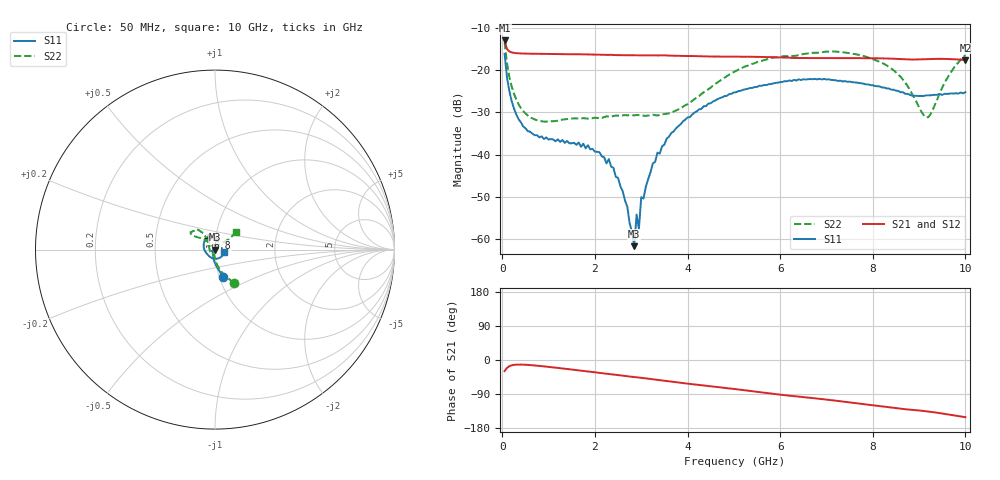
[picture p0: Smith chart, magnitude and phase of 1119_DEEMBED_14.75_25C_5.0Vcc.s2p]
!Hittite Microwave Corp.
!Digital Attenuator/PhaseShifter Rev 1.4.0
!Filename: C:\DATA\DATA\1119_DEEMBED_14.75_25C_5.0Vcc.s2p
!VNA ID: Agilent Technologies,N5224A,MY51441122,A.10.45.03
!Device type:
!2 Port Calibration.
!Temp(C): 25
!Lot Number:
!Serial Number:
!Operator:
!Misc:
!Attenuator:  14.750
# GHZ S DB R 50.0
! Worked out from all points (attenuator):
!   200 points, 50 MHz to 10 GHz, reference 50 ohm
!   highest |S21| = -12.92 dB at 50 MHz (marker M1); lowest = -17.6 dB at 10 GHz (marker M2)
!   lowest |S11| = -61.7 dB at 2.85 GHz (marker M3), VSWR 1.00, Z = 50 - j0.0816 ohm
!   |S11| at or under -10 dB: start of sweep to end of sweep
!   |S22| runs from -32.2 to -13.3 dB; largest |S21 - S12| = 0.00052
!   S11 on the Smith chart (normalised r, x): 50 MHz: 1.04, -0.32; 6.8 GHz: 0.92, +0.12; 10 GHz: 1.11, -0.03
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0.05  -16.11 -73.8  -12.92 -29.2  -12.92 -29.2  -13.31 -60.8
0.1  -21.57 -88.2  -14.94 -21.1  -14.94 -21.1  -18.22 -75.5
0.2  -27.19 -102.8  -15.74 -14.1  -15.75 -14.1  -23.73 -87.0
0.45  -33.29 -125.7  -16.02 -12.2  -16.02 -12.2  -29.64 -97.4
0.85  -35.66 -148.1  -16.10 -16.2  -16.10 -16.2  -32.09 -105.8
1.75  -37.40 -160.8  -16.21 -28.9  -16.22 -28.9  -31.36 -116.2
2.4  -43.11 -169.7  -16.37 -38.8  -16.37 -38.9  -30.85 -133.3
2.7  -52.37 -117.8  -16.43 -42.9  -16.44 -42.9  -30.70 -142.0
2.85  -61.70 -83.1  -16.44 -45.0  -16.45 -45.1  -30.70 -148.6
2.9  -54.20 -8.0  -16.46 -45.6  -16.47 -45.6  -30.59 -151.2
2.95  -57.62 -33.9  -16.44 -46.2  -16.45 -46.3  -30.64 -153.5
3  -50.09 14.6  -16.44 -47.1  -16.45 -47.1  -30.67 -156.1
3.05  -50.41 15.9  -16.45 -47.8  -16.46 -47.9  -30.75 -158.3
3.4  -39.77 45.4  -16.46 -53.0  -16.47 -53.1  -30.58 -176.3
4  -31.20 52.6  -16.62 -62.3  -16.63 -62.4  -28.07 149.8
5.05  -25.20 72.8  -16.77 -77.1  -16.79 -77.1  -20.11 125.7
6.7  -22.11 117.8  -17.08 -100.5  -17.09 -100.5  -15.85 139.8
6.8  -22.14 120.5  -17.10 -101.9  -17.11 -101.9  -15.84 141.1
8.35  -24.33 176.8  -17.22 -124.8  -17.22 -124.8  -19.18 142.5
9.2  -25.95 -110.7  -17.33 -136.0  -17.35 -136.0  -31.11 82.0
9.6  -25.61 -65.5  -17.31 -143.2  -17.33 -143.2  -22.00 38.4
10  -25.18 -16.5  -17.56 -150.9  -17.57 -150.9  -16.41 39.7
